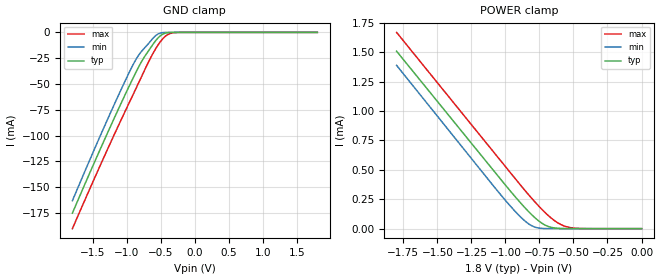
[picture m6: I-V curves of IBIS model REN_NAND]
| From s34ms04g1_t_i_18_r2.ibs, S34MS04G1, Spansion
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|   Model REN_NAND
[Model]   REN_NAND
Model_type   Input
Vinl = 0.360V
Vinh = 1.440V
| variable   typ   min   max
C_comp   2.20pF   1.98pF   2.64pF
| variable   typ   min   max
[Temperature Range]  25.00   -30.00   85.00
[Voltage Range]   1.800   1.700   1.950
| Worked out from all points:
|   GND clamp passes 1 mA (typ) near -0.44 V on its own axis
|   POWER clamp passes 1 mA (typ) near -1.44 V on its own axis
[GND_clamp]
| voltage   I(typ)   I(min)   I(max)
-1.8V     -175.3mA   -163.2mA   -190.3mA
-1.296V   -99.32mA   -86.21mA   -115.1mA
-1.044V   -63.1mA    -49.77mA   -79.22mA
-900mV    -43.2mA    -30.29mA   -59.22mA
-828mV    -33.68mA   -22.28mA   -49.15mA
-756mV    -25.26mA   -16.29mA   -39mA
-612mV    -11.24mA   -5.394mA   -19.98mA
-504mV    -3.098mA   -584uA     -8.715mA
-432mV    -701.2uA   -55.31uA   -3.643mA
-360mV    -93.94uA   -2.943uA   -1.016mA
-252mV    -2.155uA   -17.44nA   -71.48uA
1.8V      140.8pA    79.49pA    15.92nA
[POWER_clamp]
| voltage   I(typ)   I(min)   I(max)
-1.8V     1.509mA    1.389mA    1.669mA
-1.026V   407.3uA    276.2uA    565.2uA
-900mV    233.7uA    112.3uA    385.7uA
-828mV    143uA      39.64uA    286.4uA
-774mV    83.56uA    9.838uA    215.7uA
-702mV    26.52uA    788.5nA    129.8uA
-630mV    4.494uA    62.15nA    60.65uA
-558mV    538.1nA    3.703nA    18.7uA
-450mV    16.7nA     132.3pA    1.525uA
0V        0A         0A         0A
